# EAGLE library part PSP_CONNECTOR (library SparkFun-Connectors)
Connector for the PlayStation Portable (PSP) screen ribbon cable We no longer sell the screens, however we do still sell the connector. Here is the connector we sell at SparkFun: Color 24-Bit LCD 4.3" PSP Connector (LCD-08355) Datasheet
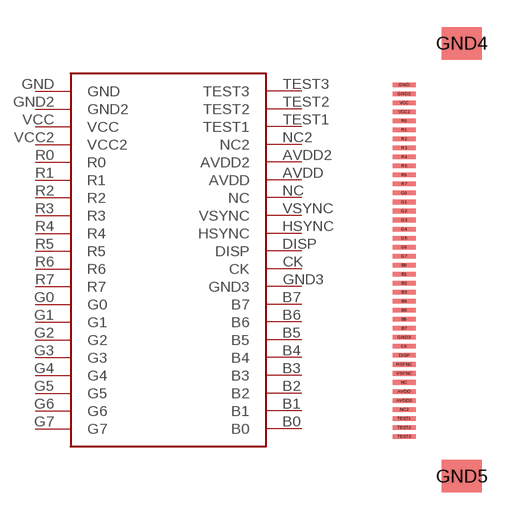
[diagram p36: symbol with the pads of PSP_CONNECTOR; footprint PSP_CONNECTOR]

Designator prefix J

## PSP_CONNECTOR (SF_ID: LCD-08355)  [PSP_CONNECTOR]
AVDD  AVDD
AVDD2  AVDD2
B0  B0
B1  B1
B2  B2
B3  B3
B4  B4
B5  B5
B6  B6
B7  B7
CK  CK
DISP  DISP
G0  G0
G1  G1
G2  G2
G3  G3
G4  G4
G5  G5
G6  G6
G7  G7
GND  GND
GND2  GND2
GND3  GND3
HSYNC  HSYNC
NC  NC
NC2  NC2
R0  R0
R1  R1
R2  R2
R3  R3
R4  R4
R5  R5
R6  R6
R7  R7
TEST1  TEST1
TEST2  TEST2
TEST3  TEST3
VCC  VCC
VCC2  VCC2
VSYNC  VSYNC

## Footprint PSP_CONNECTOR (pad centres in mm)
ZIF PSP Connector Specifications: Pin count: 42 Pin pitch:0.5mm Datasheet referenced for footprint Example device(s): PSP_CONNECTOR
smd 0.001 x 0.001 bottom: . 4.4,25.3
smd 1.27 x 0.254: AVDD 1,6; AVDD2 1,5.5; B0 1,13; B1 1,12.5; B2 1,12; B3 1,11.5; B4 1,11; B5 1,10.5; B6 1,10; B7 1,9.5; CK 1,8.5; DISP 1,8; G0 1,17; G1 1,16.5; G2 1,16; G3 1,15.5; G4 1,15; G5 1,14.5; G6 1,14; G7 1,13.5; GND 1,23; GND2 1,22.5; GND3 1,9; HSYNC 1,7.5; NC 1,6.5; NC2 1,5; R0 1,21; R1 1,20.5; R2 1,20; R3 1,19.5; R4 1,19; R5 1,18.5; R6 1,18; R7 1,17.5; TEST1 1,4.5; TEST2 1,4; TEST3 1,3.5; VCC 1,22; VCC2 1,21.5; VSYNC 1,7
smd 2.2 x 1.8: GND4 4.2,25.3; GND5 4.2,1.3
